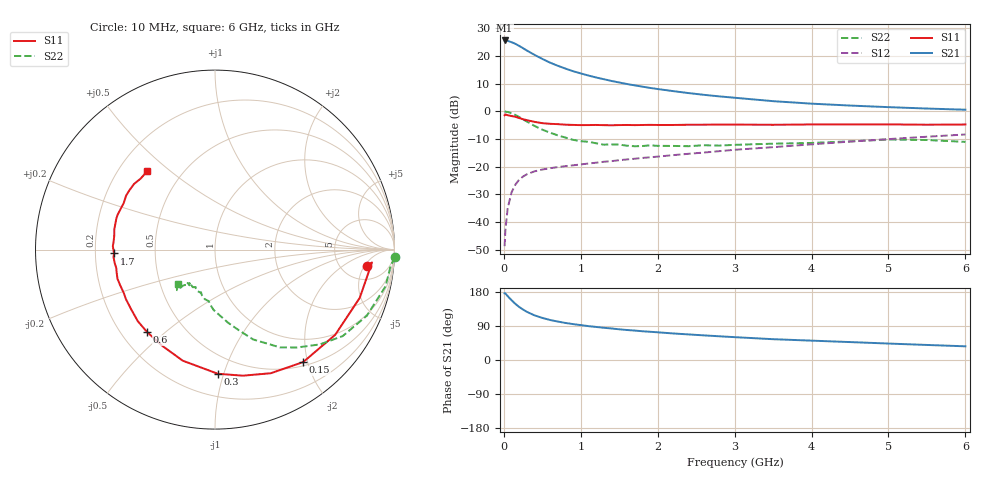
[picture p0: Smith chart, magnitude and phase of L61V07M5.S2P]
!  INFINEON TECHNOLOGIES Small Signal Semiconductors
! BFR380L3 , Si-NPN RF-Transistor in TSLP-3-1
!  Vce=1 V,  Ic=7.5 mA
! Common Emitter S-Parameters:  07. March 2005
#  GHz  S  MA  R  50
! f  S11  S21  S12  S22
! GHz  Mag  Ang  Mag  Ang  Mag  Ang  Mag  Ang
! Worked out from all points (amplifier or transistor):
!   36 points, 10 MHz to 6 GHz, reference 50 ohm
!   highest |S21| = 25.5 dB at 10 MHz (marker M1)
!   |S21| within 3 dB of that: start of sweep to 262.2 MHz
!   unconditionally stable (mu >= 1): 2.191 GHz to 4.924 GHz
!   at 250 MHz: K = 0.23, MSG = 23.1 dB, |S12| = -23.5 dB
!   at 1.4 GHz: K = 0.85, MSG = 14.5 dB, |S12| = -18.0 dB
!   at 6 GHz: K = 0.98, MSG = 4.5 dB, |S12| = -8.4 dB
!   S11 on the Smith chart (normalised r, x): 10 MHz: 9, -6; 150 MHz: 0.56, -1.92; 300 MHz: 0.36, -0.96; 600 MHz: 0.31, -0.43; 1.7 GHz: 0.28, -0.02; 6 GHz: 0.32, +0.42
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0.01  0.8492 -6.1  18.93 176.0  0.0037 84.2  1.006 -2.5
0.02  0.8775 -4.7  18.82 175.7  0.0071 90.4  0.9834 -5.0
0.05  0.8502 -18.4  18.61 168.5  0.0179 82.6  0.9723 -12.1
0.1  0.821 -35.3  17.63 157.9  0.0345 72.5  0.9229 -23.5
0.15  0.7963 -51.9  16.47 148.1  0.0477 65.0  0.8593 -34.1
0.2  0.7557 -65.7  15.06 139.8  0.0587 59.9  0.7877 -42.1
0.25  0.7196 -77.5  13.73 133.1  0.0667 54.1  0.7119 -50.0
0.3  0.6919 -88.7  12.44 127.0  0.0733 50.9  0.654 -56.4
0.4  0.6445 -106.2  10.39 117.7  0.0827 46.2  0.5439 -67.0
0.5  0.6111 -118.9  8.796 111.1  0.0891 43.6  0.4669 -73.7
0.6  0.5949 -129.6  7.545 105.6  0.0941 42.4  0.4118 -80.1
0.8  0.5733 -144.6  5.892 97.8  0.1026 42.0  0.3363 -91.3
0.9  0.568 -150.8  5.282 94.7  0.1061 42.4  0.3058 -95.2
1.1  0.5644 -159.3  4.409 89.4  0.1144 44.0  0.2819 -101.6
1.4  0.5596 -169.4  3.52 83.2  0.1262 46.2  0.2528 -109.1
1.7  0.5633 -177.8  2.936 77.7  0.1395 48.5  0.2344 -117.4
2.2  0.5666 172.3  2.311 70.1  0.162 51.8  0.2374 -122.2
2.8  0.5765 162.3  1.858 62.6  0.191 54.9  0.2406 -129.3
3.5  0.5709 152.9  1.523 54.9  0.2257 55.8  0.2607 -130.7
4.5  0.5802 145.4  1.269 47.3  0.284 57.3  0.2869 -132.4
5.5  0.5727 136.2  1.121 39.7  0.3479 55.7  0.3034 -134.4
6  0.5781 130.6  1.068 36.1  0.3821 54.1  0.2808 -137.6
